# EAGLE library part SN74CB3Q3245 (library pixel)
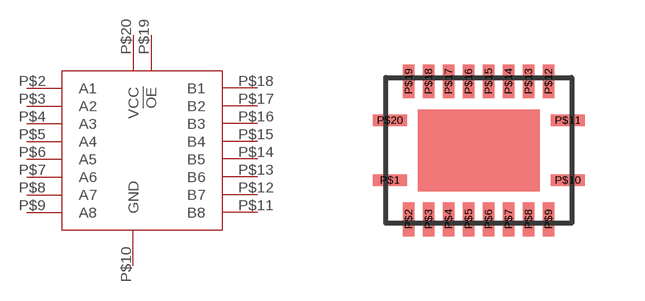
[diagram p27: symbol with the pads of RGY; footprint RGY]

Designator prefix -

## SN74CB3Q3245  [RGY]
P$2  A1
P$3  A2
P$4  A3
P$5  A4
P$6  A5
P$7  A6
P$8  A7
P$9  A8
P$10  GND
P$11  B8
P$12  B7
P$13  B6
P$14  B5
P$15  B4
P$16  B3
P$17  B2
P$18  B1
P$19  !OE
P$20  VCC

## Footprint RGY (pad centres in mm)
smd 0.85 x 0.28: P$1 -2.225,-0.75; P$10 2.225,-0.75; P$11 2.225,0.75; P$20 -2.225,0.75
smd 0.28 x 0.85: P$2 -1.75,-1.725; P$3 -1.25,-1.725; P$4 -0.75,-1.725; P$5 -0.25,-1.725; P$6 0.25,-1.725; P$7 0.75,-1.725; P$8 1.25,-1.725; P$9 1.75,-1.725; P$12 1.75,1.725; P$13 1.25,1.725; P$14 0.75,1.725; P$15 0.25,1.725; P$16 -0.25,1.725; P$17 -0.75,1.725; P$18 -1.25,1.725; P$19 -1.75,1.725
